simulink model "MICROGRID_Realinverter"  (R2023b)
settings: Solver=ode23tb  StartTime=0  StopTime=1.5  FixedStep=1e-3  RelTol=1e-5
undefined symbols (not defined in the file or in its folder): bridge, phase, pulses, Three
libraries: spsThreePhaseSeriesRLCBranchLib x11, simulink x10, spsThreePhaseVIMeasurementLib x9, slpidlib x8, spsMeanLib x8, spsabctodq0Lib x5, spsPLL3phLib x5, spsPower3phInstantaneousLib x5, spsRMSLib x5, spsCurrentMeasurementLib x4, spsDCVoltageSourceLib x4, spsPWMGenerator2LevelLib x4
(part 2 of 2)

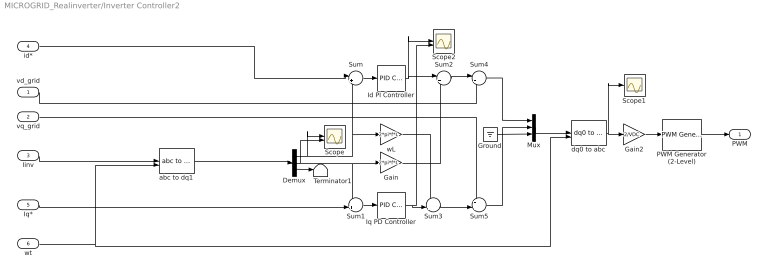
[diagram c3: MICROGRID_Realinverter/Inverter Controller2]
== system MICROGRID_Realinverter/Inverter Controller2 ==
  vd_grid : Inport
  vq_grid : Inport  Port=2
  Iinv : Inport  Port=3
  id* : Inport  Port=4
  Iq* : Inport  Port=5
  wt : Inport  Port=6
  Demux : Demux  Outputs=3
  Gain : Gain  Gain=2*pi*f*L
  Gain2 : Gain  Gain=2/VDC
  Ground : Ground
  Id PI Controller : slpidlib/PID Controller  Controller=PI  Form=Parallel  TimeDomain=Continuous-time  UseExternalTs=off  SampleTime=-1  IntegratorMethod=Forward Euler  FilterMethod=Forward Euler  ControllerParametersSource=internal  P=kp  I=ki  UseKiTs=off  D=0  N=100  UseFilter=on  TunerSelectOption=Transfer Function Based (PID Tuner App)  InitialConditionSource=internal  InitialConditionForIntegrator=0  InitialConditionForFilter=0  DifferentiatorICPrevScaledInput=0  ExternalReset=none  TrackingMode=off  Kt=1  LimitOutput=off  SatLimitsSource=internal  UpperSaturationLimit=inf  LowerSaturationLimit=-inf  LinearizeAsGain=on  AntiWindupMode=none  Kb=1  LimitIntegrator=off  UpperIntegratorSaturationLimit=inf  LowerIntegratorSaturationLimit=-inf  POutMin=[]  POutMax=[]  IOutMin=[]  IOutMax=[]  DOutMin=[]  DOutMax=[]  NOutMin=[]  NOutMax=[]  SumOutMin=[]  SumOutMax=[]  SaturationOutMin=[]  SaturationOutMax=[]  PParamMin=[]  PParamMax=[]  IParamMin=[]  IParamMax=[]  DParamMin=[]  DParamMax=[]  NParamMin=[]  NParamMax=[]  KbParamMin=[]  KbParamMax=[]  KtParamMin=[]  KtParamMax=[]  KbOutMin=[]  KbOutMax=[]  KtOutMin=[]  KtOutMax=[]  IntegratorOutMin=[]  IntegratorOutMax=[]  FilterOutMin=[]  FilterOutMax=[]  SumI1OutMin=[]  SumI1OutMax=[]  SumI2OutMin=[]  SumI2OutMax=[]  SumI3OutMin=[]  SumI3OutMax=[]  SumI4OutMin=[]  SumI4OutMax=[]  SumDOutMin=[]  SumDOutMax=[]  DifferentiatorOutMin=[]  DifferentiatorOutMax=[]  FilterDiffOutCoefMin=[]  FilterDiffOutCoefMax=[]  ReciprocalOutMin=[]  ReciprocalOutMax=[]  SumDenOutMin=[]  SumDenOutMax=[]  SumNumOutMin=[]  SumNumOutMax=[]  DivideOutMin=[]  DivideOutMax=[]  UdiffTsProdOutMin=[]  UdiffTsProdOutMax=[]  NTsProdOutMin=[]  NTsProdOutMax=[]  UintegralTsProdOutMin=[]  UintegralTsProdOutMax=[]  UngainTsProdOutMin=[]  UngainTsProdOutMax=[]  ClampingZeroOutDataTypeStr=Inherit: Inherit via back propagation  ClampingZeroOutMin=[]  ClampingZeroOutMax=[]  FilterDenConstantOutDataTypeStr=Inherit: Inherit via back propagation  FilterDenConstantOutMin=[]  FilterDenConstantOutMax=[]  PCopyOutDataTypeStr=Inherit: Inherit via back propagation  PCopyOutMin=[]  PCopyOutMax=[]  NCopyOutDataTypeStr=Inherit: Inherit via back propagation  NCopyOutMin=[]  NCopyOutMax=[]  IntegratorContinuousStateAttributes=''  IntegratorStateMustResolveToSignalObject=off  IntegratorRTWStateStorageClass=Auto  FilterContinuousStateAttributes=''  FilterStateMustResolveToSignalObject=off  FilterRTWStateStorageClass=Auto  ParallelPVariant=InternalParameters  IdealPVariant=Disabled  IVariant=InternalParameters  DVariant=Disabled  IntegratorVariant=Continuous  SatVariant=Disabled  AWVariant=Passthrough  PCopyVariant=Disabled  TRVariant=Disabled  FdbkBlocksVariant=Forward  IdealPFdbkVariant=Disabled  SatFdbkVariant=Disabled  DerivativeFilterVariant=Disabled  NVariant=Disabled  NCopyVariant=Disabled_SignalSpec  FilterICVariant=Disabled  IntegratorICVariant=InternalICs  ExternalResetVariant=Disabled  TRSumVariant=Passthrough  SumFdbkVariant=Disabled  SumVariant=Sum_PI  TsampFilterVariant=InternalTs  TsampNgainVariant=Passthrough  TsampIntegralVariant=Disabled_SignalSpec  ExternalSaturationOutDataTypeStr=Inherit: Same as second input
  Iq PD Controller : slpidlib/PID Controller  Controller=PI  Form=Parallel  TimeDomain=Continuous-time  UseExternalTs=off  SampleTime=-1  IntegratorMethod=Forward Euler  FilterMethod=Forward Euler  ControllerParametersSource=internal  P=kp  I=ki  UseKiTs=off  D=0  N=100  UseFilter=on  TunerSelectOption=Transfer Function Based (PID Tuner App)  InitialConditionSource=internal  InitialConditionForIntegrator=0  InitialConditionForFilter=0  DifferentiatorICPrevScaledInput=0  ExternalReset=none  TrackingMode=off  Kt=1  LimitOutput=off  SatLimitsSource=internal  UpperSaturationLimit=inf  LowerSaturationLimit=-inf  LinearizeAsGain=on  AntiWindupMode=none  Kb=1  LimitIntegrator=off  UpperIntegratorSaturationLimit=inf  LowerIntegratorSaturationLimit=-inf  POutMin=[]  POutMax=[]  IOutMin=[]  IOutMax=[]  DOutMin=[]  DOutMax=[]  NOutMin=[]  NOutMax=[]  SumOutMin=[]  SumOutMax=[]  SaturationOutMin=[]  SaturationOutMax=[]  PParamMin=[]  PParamMax=[]  IParamMin=[]  IParamMax=[]  DParamMin=[]  DParamMax=[]  NParamMin=[]  NParamMax=[]  KbParamMin=[]  KbParamMax=[]  KtParamMin=[]  KtParamMax=[]  KbOutMin=[]  KbOutMax=[]  KtOutMin=[]  KtOutMax=[]  IntegratorOutMin=[]  IntegratorOutMax=[]  FilterOutMin=[]  FilterOutMax=[]  SumI1OutMin=[]  SumI1OutMax=[]  SumI2OutMin=[]  SumI2OutMax=[]  SumI3OutMin=[]  SumI3OutMax=[]  SumI4OutMin=[]  SumI4OutMax=[]  SumDOutMin=[]  SumDOutMax=[]  DifferentiatorOutMin=[]  DifferentiatorOutMax=[]  FilterDiffOutCoefMin=[]  FilterDiffOutCoefMax=[]  ReciprocalOutMin=[]  ReciprocalOutMax=[]  SumDenOutMin=[]  SumDenOutMax=[]  SumNumOutMin=[]  SumNumOutMax=[]  DivideOutMin=[]  DivideOutMax=[]  UdiffTsProdOutMin=[]  UdiffTsProdOutMax=[]  NTsProdOutMin=[]  NTsProdOutMax=[]  UintegralTsProdOutMin=[]  UintegralTsProdOutMax=[]  UngainTsProdOutMin=[]  UngainTsProdOutMax=[]  ClampingZeroOutDataTypeStr=Inherit: Inherit via back propagation  ClampingZeroOutMin=[]  ClampingZeroOutMax=[]  FilterDenConstantOutDataTypeStr=Inherit: Inherit via back propagation  FilterDenConstantOutMin=[]  FilterDenConstantOutMax=[]  PCopyOutDataTypeStr=Inherit: Inherit via back propagation  PCopyOutMin=[]  PCopyOutMax=[]  NCopyOutDataTypeStr=Inherit: Inherit via back propagation  NCopyOutMin=[]  NCopyOutMax=[]  IntegratorContinuousStateAttributes=''  IntegratorStateMustResolveToSignalObject=off  IntegratorRTWStateStorageClass=Auto  FilterContinuousStateAttributes=''  FilterStateMustResolveToSignalObject=off  FilterRTWStateStorageClass=Auto  ParallelPVariant=InternalParameters  IdealPVariant=Disabled  IVariant=InternalParameters  DVariant=Disabled  IntegratorVariant=Continuous  SatVariant=Disabled  AWVariant=Passthrough  PCopyVariant=Disabled  TRVariant=Disabled  FdbkBlocksVariant=Forward  IdealPFdbkVariant=Disabled  SatFdbkVariant=Disabled  DerivativeFilterVariant=Disabled  NVariant=Disabled  NCopyVariant=Disabled_SignalSpec  FilterICVariant=Disabled  IntegratorICVariant=InternalICs  ExternalResetVariant=Disabled  TRSumVariant=Passthrough  SumFdbkVariant=Disabled  SumVariant=Sum_PI  TsampFilterVariant=InternalTs  TsampNgainVariant=Passthrough  TsampIntegralVariant=Disabled_SignalSpec  ExternalSaturationOutDataTypeStr=Inherit: Same as second input
  Mux : Mux  Inputs=3
  PWM Generator (2-Level) : spsPWMGenerator2LevelLib/PWM Generator (2-Level)  ModulatorType=Three-phase bridge (6 pulses)  ModulatorMode=Unsynchronized  Fc=fsw  Pc=0  nF=27  MinMax="[ -1  1 ]"  SamplingTechnique=Natural  ModulatingSignals=off  m=0.8  Freq=60  Phase=0  Ts=0  ShowCarrierOutport=off
  Scope : Scope  NumInputPorts=2
  Scope1 : Scope
  Scope2 : Scope  NumInputPorts=2
  Sum : Sum  Inputs=|+-
  Sum1 : Sum  Inputs=-+|
  Sum2 : Sum  Inputs=|++
  Sum3 : Sum  Inputs=-+|
  Sum4 : Sum  Inputs=|++
  Sum5 : Sum  Inputs=++|
  Terminator1 : Terminator
  abc to dq1 : spsabctodq0Lib/abc to dq0  Alignment=90 degrees behind phase A axis
  dq0 to abc : spsdq0toabcLib/dq0 to abc  Alignment=90 degrees behind phase A axis
  wL : Gain  Gain=2*pi*f*L
  PWM : Outport
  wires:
  PWM Generator (2-Level)/1 -> PWM/1
  Id PI Controller/1 -> Scope2/1, Sum2/1
  Gain2/1 -> PWM Generator (2-Level)/1
  Ground/1 -> Mux/3
  wL/1 -> Sum3/1
  Gain/1 -> Sum2/2
  dq0 to abc/1 -> Scope1/1, Gain2/1
  vd_grid/1 -> Sum4/2
  Sum1/1 -> Iq PD Controller/1
  Sum/1 -> Id PI Controller/1
  abc to dq1/1 -> Demux/1
  Sum2/1 -> Sum4/1
  Mux/1 -> dq0 to abc/1
  vq_grid/1 -> Sum5/1
  Sum3/1 -> Sum5/2
  Sum5/1 -> Mux/2
  Demux/1 -> Scope/1, Sum/2, wL/1
  Iq PD Controller/1 -> Scope2/2, Sum3/2
  Sum4/1 -> Mux/1
  Demux/2 -> Sum1/1, Gain/1, Scope/2
  Demux/3 -> Terminator1/1
  Iinv/1 -> abc to dq1/1
  Iq*/1 -> Sum1/2
  id*/1 -> Sum/1
  wt/1 -> abc to dq1/2, dq0 to abc/2

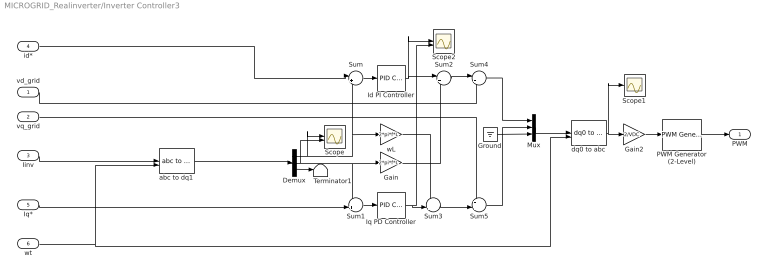
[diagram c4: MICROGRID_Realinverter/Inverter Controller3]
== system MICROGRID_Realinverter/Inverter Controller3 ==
  vd_grid : Inport
  vq_grid : Inport  Port=2
  Iinv : Inport  Port=3
  id* : Inport  Port=4
  Iq* : Inport  Port=5
  wt : Inport  Port=6
  Demux : Demux  Outputs=3
  Gain : Gain  Gain=2*pi*f*L
  Gain2 : Gain  Gain=2/VDC
  Ground : Ground
  Id PI Controller : slpidlib/PID Controller  Controller=PI  Form=Parallel  TimeDomain=Continuous-time  UseExternalTs=off  SampleTime=-1  IntegratorMethod=Forward Euler  FilterMethod=Forward Euler  ControllerParametersSource=internal  P=kp  I=ki  UseKiTs=off  D=0  N=100  UseFilter=on  TunerSelectOption=Transfer Function Based (PID Tuner App)  InitialConditionSource=internal  InitialConditionForIntegrator=0  InitialConditionForFilter=0  DifferentiatorICPrevScaledInput=0  ExternalReset=none  TrackingMode=off  Kt=1  LimitOutput=off  SatLimitsSource=internal  UpperSaturationLimit=inf  LowerSaturationLimit=-inf  LinearizeAsGain=on  AntiWindupMode=none  Kb=1  LimitIntegrator=off  UpperIntegratorSaturationLimit=inf  LowerIntegratorSaturationLimit=-inf  POutMin=[]  POutMax=[]  IOutMin=[]  IOutMax=[]  DOutMin=[]  DOutMax=[]  NOutMin=[]  NOutMax=[]  SumOutMin=[]  SumOutMax=[]  SaturationOutMin=[]  SaturationOutMax=[]  PParamMin=[]  PParamMax=[]  IParamMin=[]  IParamMax=[]  DParamMin=[]  DParamMax=[]  NParamMin=[]  NParamMax=[]  KbParamMin=[]  KbParamMax=[]  KtParamMin=[]  KtParamMax=[]  KbOutMin=[]  KbOutMax=[]  KtOutMin=[]  KtOutMax=[]  IntegratorOutMin=[]  IntegratorOutMax=[]  FilterOutMin=[]  FilterOutMax=[]  SumI1OutMin=[]  SumI1OutMax=[]  SumI2OutMin=[]  SumI2OutMax=[]  SumI3OutMin=[]  SumI3OutMax=[]  SumI4OutMin=[]  SumI4OutMax=[]  SumDOutMin=[]  SumDOutMax=[]  DifferentiatorOutMin=[]  DifferentiatorOutMax=[]  FilterDiffOutCoefMin=[]  FilterDiffOutCoefMax=[]  ReciprocalOutMin=[]  ReciprocalOutMax=[]  SumDenOutMin=[]  SumDenOutMax=[]  SumNumOutMin=[]  SumNumOutMax=[]  DivideOutMin=[]  DivideOutMax=[]  UdiffTsProdOutMin=[]  UdiffTsProdOutMax=[]  NTsProdOutMin=[]  NTsProdOutMax=[]  UintegralTsProdOutMin=[]  UintegralTsProdOutMax=[]  UngainTsProdOutMin=[]  UngainTsProdOutMax=[]  ClampingZeroOutDataTypeStr=Inherit: Inherit via back propagation  ClampingZeroOutMin=[]  ClampingZeroOutMax=[]  FilterDenConstantOutDataTypeStr=Inherit: Inherit via back propagation  FilterDenConstantOutMin=[]  FilterDenConstantOutMax=[]  PCopyOutDataTypeStr=Inherit: Inherit via back propagation  PCopyOutMin=[]  PCopyOutMax=[]  NCopyOutDataTypeStr=Inherit: Inherit via back propagation  NCopyOutMin=[]  NCopyOutMax=[]  IntegratorContinuousStateAttributes=''  IntegratorStateMustResolveToSignalObject=off  IntegratorRTWStateStorageClass=Auto  FilterContinuousStateAttributes=''  FilterStateMustResolveToSignalObject=off  FilterRTWStateStorageClass=Auto  ParallelPVariant=InternalParameters  IdealPVariant=Disabled  IVariant=InternalParameters  DVariant=Disabled  IntegratorVariant=Continuous  SatVariant=Disabled  AWVariant=Passthrough  PCopyVariant=Disabled  TRVariant=Disabled  FdbkBlocksVariant=Forward  IdealPFdbkVariant=Disabled  SatFdbkVariant=Disabled  DerivativeFilterVariant=Disabled  NVariant=Disabled  NCopyVariant=Disabled_SignalSpec  FilterICVariant=Disabled  IntegratorICVariant=InternalICs  ExternalResetVariant=Disabled  TRSumVariant=Passthrough  SumFdbkVariant=Disabled  SumVariant=Sum_PI  TsampFilterVariant=InternalTs  TsampNgainVariant=Passthrough  TsampIntegralVariant=Disabled_SignalSpec  ExternalSaturationOutDataTypeStr=Inherit: Same as second input
  Iq PD Controller : slpidlib/PID Controller  Controller=PI  Form=Parallel  TimeDomain=Continuous-time  UseExternalTs=off  SampleTime=-1  IntegratorMethod=Forward Euler  FilterMethod=Forward Euler  ControllerParametersSource=internal  P=kp  I=ki  UseKiTs=off  D=0  N=100  UseFilter=on  TunerSelectOption=Transfer Function Based (PID Tuner App)  InitialConditionSource=internal  InitialConditionForIntegrator=0  InitialConditionForFilter=0  DifferentiatorICPrevScaledInput=0  ExternalReset=none  TrackingMode=off  Kt=1  LimitOutput=off  SatLimitsSource=internal  UpperSaturationLimit=inf  LowerSaturationLimit=-inf  LinearizeAsGain=on  AntiWindupMode=none  Kb=1  LimitIntegrator=off  UpperIntegratorSaturationLimit=inf  LowerIntegratorSaturationLimit=-inf  POutMin=[]  POutMax=[]  IOutMin=[]  IOutMax=[]  DOutMin=[]  DOutMax=[]  NOutMin=[]  NOutMax=[]  SumOutMin=[]  SumOutMax=[]  SaturationOutMin=[]  SaturationOutMax=[]  PParamMin=[]  PParamMax=[]  IParamMin=[]  IParamMax=[]  DParamMin=[]  DParamMax=[]  NParamMin=[]  NParamMax=[]  KbParamMin=[]  KbParamMax=[]  KtParamMin=[]  KtParamMax=[]  KbOutMin=[]  KbOutMax=[]  KtOutMin=[]  KtOutMax=[]  IntegratorOutMin=[]  IntegratorOutMax=[]  FilterOutMin=[]  FilterOutMax=[]  SumI1OutMin=[]  SumI1OutMax=[]  SumI2OutMin=[]  SumI2OutMax=[]  SumI3OutMin=[]  SumI3OutMax=[]  SumI4OutMin=[]  SumI4OutMax=[]  SumDOutMin=[]  SumDOutMax=[]  DifferentiatorOutMin=[]  DifferentiatorOutMax=[]  FilterDiffOutCoefMin=[]  FilterDiffOutCoefMax=[]  ReciprocalOutMin=[]  ReciprocalOutMax=[]  SumDenOutMin=[]  SumDenOutMax=[]  SumNumOutMin=[]  SumNumOutMax=[]  DivideOutMin=[]  DivideOutMax=[]  UdiffTsProdOutMin=[]  UdiffTsProdOutMax=[]  NTsProdOutMin=[]  NTsProdOutMax=[]  UintegralTsProdOutMin=[]  UintegralTsProdOutMax=[]  UngainTsProdOutMin=[]  UngainTsProdOutMax=[]  ClampingZeroOutDataTypeStr=Inherit: Inherit via back propagation  ClampingZeroOutMin=[]  ClampingZeroOutMax=[]  FilterDenConstantOutDataTypeStr=Inherit: Inherit via back propagation  FilterDenConstantOutMin=[]  FilterDenConstantOutMax=[]  PCopyOutDataTypeStr=Inherit: Inherit via back propagation  PCopyOutMin=[]  PCopyOutMax=[]  NCopyOutDataTypeStr=Inherit: Inherit via back propagation  NCopyOutMin=[]  NCopyOutMax=[]  IntegratorContinuousStateAttributes=''  IntegratorStateMustResolveToSignalObject=off  IntegratorRTWStateStorageClass=Auto  FilterContinuousStateAttributes=''  FilterStateMustResolveToSignalObject=off  FilterRTWStateStorageClass=Auto  ParallelPVariant=InternalParameters  IdealPVariant=Disabled  IVariant=InternalParameters  DVariant=Disabled  IntegratorVariant=Continuous  SatVariant=Disabled  AWVariant=Passthrough  PCopyVariant=Disabled  TRVariant=Disabled  FdbkBlocksVariant=Forward  IdealPFdbkVariant=Disabled  SatFdbkVariant=Disabled  DerivativeFilterVariant=Disabled  NVariant=Disabled  NCopyVariant=Disabled_SignalSpec  FilterICVariant=Disabled  IntegratorICVariant=InternalICs  ExternalResetVariant=Disabled  TRSumVariant=Passthrough  SumFdbkVariant=Disabled  SumVariant=Sum_PI  TsampFilterVariant=InternalTs  TsampNgainVariant=Passthrough  TsampIntegralVariant=Disabled_SignalSpec  ExternalSaturationOutDataTypeStr=Inherit: Same as second input
  Mux : Mux  Inputs=3
  PWM Generator (2-Level) : spsPWMGenerator2LevelLib/PWM Generator (2-Level)  ModulatorType=Three-phase bridge (6 pulses)  ModulatorMode=Unsynchronized  Fc=fsw  Pc=0  nF=27  MinMax="[ -1  1 ]"  SamplingTechnique=Natural  ModulatingSignals=off  m=0.8  Freq=60  Phase=0  Ts=0  ShowCarrierOutport=off
  Scope : Scope  NumInputPorts=2
  Scope1 : Scope
  Scope2 : Scope  NumInputPorts=2
  Sum : Sum  Inputs=|+-
  Sum1 : Sum  Inputs=-+|
  Sum2 : Sum  Inputs=|++
  Sum3 : Sum  Inputs=-+|
  Sum4 : Sum  Inputs=|++
  Sum5 : Sum  Inputs=++|
  Terminator1 : Terminator
  abc to dq1 : spsabctodq0Lib/abc to dq0  Alignment=90 degrees behind phase A axis
  dq0 to abc : spsdq0toabcLib/dq0 to abc  Alignment=90 degrees behind phase A axis
  wL : Gain  Gain=2*pi*f*L
  PWM : Outport
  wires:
  PWM Generator (2-Level)/1 -> PWM/1
  Id PI Controller/1 -> Scope2/1, Sum2/1
  Gain2/1 -> PWM Generator (2-Level)/1
  Ground/1 -> Mux/3
  wL/1 -> Sum3/1
  Gain/1 -> Sum2/2
  dq0 to abc/1 -> Scope1/1, Gain2/1
  vd_grid/1 -> Sum4/2
  Sum1/1 -> Iq PD Controller/1
  Sum/1 -> Id PI Controller/1
  abc to dq1/1 -> Demux/1
  Sum2/1 -> Sum4/1
  Mux/1 -> dq0 to abc/1
  vq_grid/1 -> Sum5/1
  Sum3/1 -> Sum5/2
  Sum5/1 -> Mux/2
  Demux/1 -> Scope/1, Sum/2, wL/1
  Iq PD Controller/1 -> Scope2/2, Sum3/2
  Sum4/1 -> Mux/1
  Demux/2 -> Sum1/1, Gain/1, Scope/2
  Demux/3 -> Terminator1/1
  Iinv/1 -> abc to dq1/1
  Iq*/1 -> Sum1/2
  id*/1 -> Sum/1
  wt/1 -> abc to dq1/2, dq0 to abc/2

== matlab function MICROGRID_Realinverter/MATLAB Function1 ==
function [Id1,Id,Iq1,Iq,sign] = current (Pe,Qe,Vd_grid,Vq_grid,Fault)

if Pe <=0
    Pes=Fault*Pe;
else 
    Pes=Pe;
end
sign=Pes/(abs(Pes));
Id=666.6666667*(Vd_grid*Pes+Vq_grid*Qe)/((Vd_grid^2)+(Vq_grid^2));
Iq=666.6666667*(Vq_grid*Pes-Vd_grid*Qe)/((Vd_grid^2)+(Vq_grid^2));
tang=Qe/Pes;
Id1=sqrt(20416.666666666666/(1+(tang^2)));
Iq1=abs(Id1*tang);

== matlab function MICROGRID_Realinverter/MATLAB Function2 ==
function [Id1,Id,Iq1,Iq] = current (Pe,Qe,Vd_grid,Vq_grid)

Id=666.6666667*(Vd_grid*Pe+Vq_grid*Qe)/((Vd_grid^2)+(Vq_grid^2));
Iq=666.6666667*(Vq_grid*Pe-Vd_grid*Qe)/((Vd_grid^2)+(Vq_grid^2));
tang=Qe/Pe;
Id1=sqrt(46207.9999997/(1+(tang^2)));
Iq1=abs(Id1*tang);

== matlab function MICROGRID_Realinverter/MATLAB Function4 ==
function [Id1,Id,Iq1,Iq] = current (Pe,Qe,Vd_grid,Vq_grid)

Id=666.6666667*(Vd_grid*Pe+Vq_grid*Qe)/((Vd_grid^2)+(Vq_grid^2));
Iq=666.6666667*(Vq_grid*Pe-Vd_grid*Qe)/((Vd_grid^2)+(Vq_grid^2));
tang=Qe/Pe;
Id1=sqrt(352799.999998/(1+(tang^2)));
Iq1=abs(Id1*tang);

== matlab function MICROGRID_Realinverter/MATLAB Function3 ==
function [Id1,Id,Iq1,Iq] = current (Pe,Qe,Vd_grid,Vq_grid)

Id=666.6666667*(Vd_grid*Pe+Vq_grid*Qe)/((Vd_grid^2)+(Vq_grid^2));
Iq=666.6666667*(Vq_grid*Pe-Vd_grid*Qe)/((Vd_grid^2)+(Vq_grid^2));
tang=Qe/Pe;
Id1=sqrt(352799.999998/(1+(tang^2)));
Iq1=abs(Id1*tang);
